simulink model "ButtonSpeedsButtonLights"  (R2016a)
settings: Solver=FixedStepAuto  StartTime=0.0  StopTime=inf  RelTol=1e-3
libraries: miniQ x3

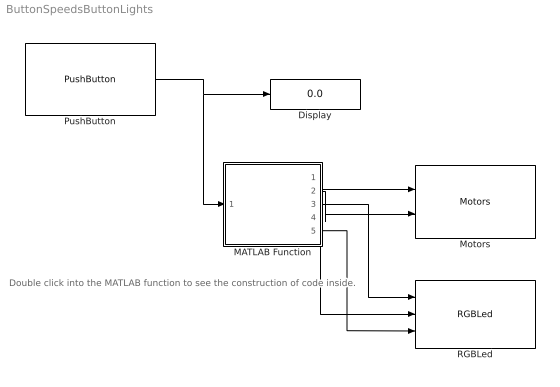
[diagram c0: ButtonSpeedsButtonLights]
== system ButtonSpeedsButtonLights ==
  note: Double click into the MATLAB function to see the construction of code inside.
  Display : Display
  MATLAB Function : MATLAB Function  TreatAsAtomicUnit=on
  Motors : miniQ/Motors  flipLeft=off  flipRight=off
  PushButton : miniQ/PushButton  sampleTime_dd=0.1  debug_dd=off
  RGBLed : miniQ/RGBLed
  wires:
  PushButton/1 -> Display/1, MATLAB Function/1(button)
  MATLAB Function/1(motor1) -> Motors/1
  MATLAB Function/2(motor2) -> Motors/2
  MATLAB Function/3(red) -> RGBLed/1
  MATLAB Function/4(green) -> RGBLed/2
  MATLAB Function/5(blue) -> RGBLed/3

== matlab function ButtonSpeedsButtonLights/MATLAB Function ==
function [motor1,motor2,red,green,blue] = fcn(button)

if button == 1
    motor1=40;
    motor2=40;
    
    red=0;
    green=255;
    blue=0;
    
else if button == 2
    motor1=130;
    motor2=130;
    
    red=255;
    green=0;
    blue=0;
    
    else if button ==3
        motor1=255;
        motor2=255;
            
        red=0;
        green=0;
        blue=255;

else
    motor1=0;
    motor2=0;
    
    red=0;
    green=0;
    blue=0;
        end
    end
end
end
